| IBIS file stm32u073_083_ufqfpn48.ibs
[IBIS ver] 4.2
[File name] stm32u073_083_ufqfpn48.ibs
[File Rev] 0.3
[Date] 20-02-2024
[Source] Data Created at STMicroelectronics
[Notes]  File originated from ELDO simulations.
[Disclaimer]  This information is for modeling purpose only and is
   not guaranteed. The information is subject to change without
   notice.
[Copyright] Copyright 2024 STMicroelectronics Inc.
|   Component stm32u073_083_ufqfpn48
[Component] stm32u073_083_ufqfpn48
[Manufacturer] STMicroelectronics
[Package]
| variable   typ   min   max
R_pkg  0  NA  NA
L_pkg  0  NA  NA
C_pkg  0  NA  NA
[Pin]   signal_name   model_name
1  VBAT  power
2  PC13  io8_ft_v33
3  PC14-OSC32_IN  io8_ft_v33
4  PC15-OSC32_OUT  io8_ft
5  PF0-OSC_IN  io8_ft
6  PF1-OSC_OUT  io8_ft
7  PF2-NRST  ioreset_ft_v33
8  VSSA_VREFM  nc
9  VDDA_VREFP  nc
10  PA0  io8_ft_v33
11  PA1  io8_ft_v33
12  PA2  io8_ft_v33
13  PA3  io8_ft
14  PA4  io8_ft
15  PA5  io8_ft
16  PA6  io8_ft_i2c
17  PA7  io8_ft_i2c
18  PB0  io8_ft
19  PB1  io8_ft
20  PB2  io8_ft
21  PB10  io8_ft_i2c
22  PB11  io8_ft_i2c
23  VSS  gnd
24  VDD  power
25  PB12  io8_ft
26  PB13  io8_ft_i2c
27  PB14  io8_ft_i2c
28  PB15  io8_ft_v33
29  PA8  io8_ft
30  PA9  io8_ft_i2c
31  PA10  io8_ft_i2c
32  PA11  io8usb_ft_phy
33  PA12  io8usb_ft_phy
34  PA13  io8_ft
35  VSS  gnd
36  VDDUSB  power
37  PA14  io8_ft
38  PA15  io8_ft
39  PB3  io8_ft_i2c
40  PB4  io8_ft_i2c
41  PB5  io8_ft
42  PB6  io8_ft_i2c
43  PB7  io8_ft_i2c
44  PF3-BOOT0  io8_ft_v33
45  PB8  io8_ft_i2c
46  PB9  io8_ft_i2c
47  VSS  gnd
48  VDD  power
[Package Model]   489-qfpn-7x7-48-ldo-240125
[Pin Mapping]   pulldown_ref   pullup_ref   | Comment
1  nc  vsw
2  gndio  vddio  | Depending on IO usage
| 2  gndio  vsw  | Depending on IO usage
3  gndio  vddio  | Depending on IO usage
| 3  gndio  vsw  | Depending on IO usage
4  gndio  vddio  | Depending on IO usage
| 4  gndio  vsw  | Depending on IO usage
5  gndio  vddio
6  gndio  vddio
7  gndio  vddio
8  nc  nc
9  nc  nc
10  gndio  vddio
11  gndio  vddio
12  gndio  vddio
13  gndio  vddio
14  gndio  vddio
15  gndio  vddio
16  gndio  vddio
17  gndio  vddio
18  gndio  vddio
19  gndio  vddio
20  gndio  vddio
21  gndio  vddio
22  gndio  vddio
23  gndio  nc
24  nc  vddio
25  gndio  vddio
26  gndio  vddio
27  gndio  vddio
28  gndio  vddio
29  gndio  vddio
30  gndio  vddio
31  gndio  vddio
32  gndio  vddusb  | Depending on IO usage
| 32  gndio  vddio  | Depending on IO usage
33  gndio  vddusb  | Depending on IO usage
| 33  gndio  vddio  | Depending on IO usage
34  gndio  vddio
35  gndio  nc
36  nc  vddusb
37  gndio  vddio
38  gndio  vddio
39  gndio  vddio
40  gndio  vddio
41  gndio  vddio
42  gndio  vddio
43  gndio  vddio
44  gndio  vddio
45  gndio  vddio
46  gndio  vddio
47  gndio  nc
48  nc  vddio
|[Diff Pin]  inv_pin  vdiff  tdelay_typ  tdelay_min  tdelay_max
|33  32  NA  NA  NA  NA
[Model Selector] io8_ft
io8_ft_ls_1v2   "GPIO - 5V tolerant - 1.2V range - Low speed"
io8_ft_ms_1v2   "GPIO - 5V tolerant - 1.2V range - Med speed"
io8_ft_fs_1v2   "GPIO - 5V tolerant - 1.2V range - Fast speed"
io8_ft_hs_1v2   "GPIO - 5V tolerant - 1.2V range - High speed"
io8_ft_ls_1v8   "GPIO - 5V tolerant - 1.8V range - Low speed"
io8_ft_ms_1v8   "GPIO - 5V tolerant - 1.8V range - Med speed"
io8_ft_fs_1v8   "GPIO - 5V tolerant - 1.8V range - Fast speed"
io8_ft_hs_1v8   "GPIO - 5V tolerant - 1.8V range - High speed"
io8_ft_ls_3v3   "GPIO - 5V tolerant - 3.3V range - Low speed"
io8_ft_ms_3v3   "GPIO - 5V tolerant - 3.3V range - Med speed"
io8_ft_fs_3v3   "GPIO - 5V tolerant - 3.3V range - Fast speed"
io8_ft_hs_3v3   "GPIO - 5V tolerant - 3.3V range - High speed"
[Model Selector] io8_ft_i2c
io8_ft_ls_1v2   "GPIO - 5V tolerant - 1.2V range - Low speed"
io8_ft_ms_1v2   "GPIO - 5V tolerant - 1.2V range - Med speed"
io8_ft_fs_1v2   "GPIO - 5V tolerant - 1.2V range - Fast speed"
io8_ft_hs_1v2   "GPIO - 5V tolerant - 1.2V range - High speed"
io8_ft_ls_1v8   "GPIO - 5V tolerant - 1.8V range - Low speed"
io8_ft_ms_1v8   "GPIO - 5V tolerant - 1.8V range - Med speed"
io8_ft_fs_1v8   "GPIO - 5V tolerant - 1.8V range - Fast speed"
io8_ft_hs_1v8   "GPIO - 5V tolerant - 1.8V range - High speed"
io8_ft_ls_3v3   "GPIO - 5V tolerant - 3.3V range - Low speed"
io8_ft_ms_3v3   "GPIO - 5V tolerant - 3.3V range - Med speed"
io8_ft_fs_3v3   "GPIO - 5V tolerant - 3.3V range - Fast speed"
io8_ft_hs_3v3   "GPIO - 5V tolerant - 3.3V range - High speed"
io8_ft_i2c_ls_1v2   "GPIO I2C open-drain - 5V tolerant - 1.2V range - Low speed"
io8_ft_i2c_ms_1v2   "GPIO I2C open-drain - 5V tolerant - 1.2V range - Med speed"
io8_ft_i2c_fs_1v2   "GPIO I2C open-drain - 5V tolerant - 1.2V range - Fast speed"
io8_ft_i2c_hs_1v2   "GPIO I2C open-drain - 5V tolerant - 1.2V range - High speed"
io8_ft_i2c_ls_1v8   "GPIO I2C open-drain - 5V tolerant - 1.8V range - Low speed"
io8_ft_i2c_ms_1v8   "GPIO I2C open-drain - 5V tolerant - 1.8V range - Med speed"
io8_ft_i2c_fs_1v8   "GPIO I2C open-drain - 5V tolerant - 1.8V range - Fast speed"
io8_ft_i2c_hs_1v8   "GPIO I2C open-drain - 5V tolerant - 1.8V range - High speed"
io8_ft_i2c_ls_3v3   "GPIO I2C open-drain - 5V tolerant - 3.3V range - Low speed"
io8_ft_i2c_ms_3v3   "GPIO I2C open-drain - 5V tolerant - 3.3V range - Med speed"
io8_ft_i2c_fs_3v3   "GPIO I2C open-drain - 5V tolerant - 3.3V range - Fast speed"
io8_ft_i2c_hs_3v3   "GPIO I2C open-drain - 5V tolerant - 3.3V range - High speed"
io8_ft_i2c_fmp_3v3   "GPIO I2C open-drain fm+ - 5V tolerant - 3.3V range"
[Model Selector] io8_ft_v33
io8_ft_v33_ls_1v2   "GPIO_V33 - 5V tolerant - 1.2V range - Low speed"
io8_ft_v33_ms_1v2   "GPIO_V33 - 5V tolerant - 1.2V range - Med speed"
io8_ft_v33_fs_1v2   "GPIO_V33 - 5V tolerant - 1.2V range - Fast speed"
io8_ft_v33_hs_1v2   "GPIO_V33 - 5V tolerant - 1.2V range - High speed"
io8_ft_v33_ls_1v8   "GPIO_V33 - 5V tolerant - 1.8V range - Low speed"
io8_ft_v33_ms_1v8   "GPIO_V33 - 5V tolerant - 1.8V range - Med speed"
io8_ft_v33_fs_1v8   "GPIO_V33 - 5V tolerant - 1.8V range - Fast speed"
io8_ft_v33_hs_1v8   "GPIO_V33 - 5V tolerant - 1.8V range - High speed"
io8_ft_v33_ls_3v3   "GPIO_V33 - 5V tolerant - 3.3V range - Low speed"
io8_ft_v33_ms_3v3   "GPIO_V33 - 5V tolerant - 3.3V range - Med speed"
io8_ft_v33_fs_3v3   "GPIO_V33 - 5V tolerant - 3.3V range - Fast speed"
io8_ft_v33_hs_3v3   "GPIO_V33 - 5V tolerant - 3.3V range - High speed"
[Model Selector] io8usb_ft_phy
io8_ft_ls_1v2   "GPIO - 5V tolerant - 1.2V range - Low speed"
io8_ft_ms_1v2   "GPIO - 5V tolerant - 1.2V range - Med speed"
io8_ft_fs_1v2   "GPIO - 5V tolerant - 1.2V range - Fast speed"
io8_ft_hs_1v2   "GPIO - 5V tolerant - 1.2V range - High speed"
io8_ft_ls_1v8   "GPIO - 5V tolerant - 1.8V range - Low speed"
io8_ft_ms_1v8   "GPIO - 5V tolerant - 1.8V range - Med speed"
io8_ft_fs_1v8   "GPIO - 5V tolerant - 1.8V range - Fast speed"
io8_ft_hs_1v8   "GPIO - 5V tolerant - 1.8V range - High speed"
io8_ft_ls_3v3   "GPIO - 5V tolerant - 3.3V range - Low speed"
io8_ft_ms_3v3   "GPIO - 5V tolerant - 3.3V range - Med speed"
io8_ft_fs_3v3   "GPIO - 5V tolerant - 3.3V range - Fast speed"
io8_ft_hs_3v3   "GPIO - 5V tolerant - 3.3V range - High speed"
io8usb_ft_phy_hs_3v3   "USB full speed"
io8usb_ft_phy_ls_3v3   "USB low speed"
[Model Selector] ioreset_ft_v33
ioreset_ft_v33_1v2   "Reset PAD. 5V tolerant. 1.2V range"
ioreset_ft_v33_1v8   "Reset PAD. 5V tolerant. 1.8V range"
ioreset_ft_v33_3v3   "Reset PAD. 5V tolerant. 3.3V range"
[Define Package Model]  489-qfpn-7x7-48-ldo-240125
[Manufacturer]  Unknown
[OEM]  Unknown
[Description]  None
[Number Of Pins]  46
[Pin Numbers]
| Pin Num   Terminal Name
10 | PA0
11 | PA1
12 | PA2
13 | PA3
14 | PA4
15 | PA5
16 | PA6
17 | PA7
29 | PA8
30 | PA9
31 | PA10
32 | PA11
33 | PA12
34 | PA13
37 | PA14
38 | PA15
18 | PB0
19 | PB1
20 | PB2
39 | PB3
40 | PB4
41 | PB5
42 | PB6
43 | PB7
45 | PB8
46 | PB9
21 | PB10
22 | PB11
25 | PB12
26 | PB13
27 | PB14
28 | PB15
2 | PC13
3 | PC14-OSC32_IN
4 | PC15-OSC32_OUT
5 | PF0-OSC_IN
6 | PF1-OSC_OUT
7 | PF2-NRST
44 | PF3-BOOT0
1 | VBAT
48 | VDD
24 | VDD
9 | VDDA_VREFP
36 | VDDUSB
23 | VSS
8 | VSSA_VREFM
|[Merged Pins]  23
|35  |  VSS
|47  |  VSS
[Model Data]
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[End Model Data]
[End Package Model]
|End [Component]
| Models and submodels in the file (42): io8_ft_fs_1v2 (I/O), io8_ft_fs_1v8 (I/O), io8_ft_fs_3v3 (I/O), io8_ft_hs_1v2 (I/O), io8_ft_hs_1v8 (I/O), io8_ft_hs_3v3 (I/O), io8_ft_i2c_fmp_3v3 (I/O_open_drain), io8_ft_i2c_fs_1v2 (I/O_open_drain), io8_ft_i2c_fs_1v8 (I/O_open_drain), io8_ft_i2c_fs_3v3 (I/O_open_drain), io8_ft_i2c_hs_1v2 (I/O_open_drain), io8_ft_i2c_hs_1v8 (I/O_open_drain), io8_ft_i2c_hs_3v3 (I/O_open_drain), io8_ft_i2c_ls_1v2 (I/O_open_drain), io8_ft_i2c_ls_1v8 (I/O_open_drain), io8_ft_i2c_ls_3v3 (I/O_open_drain), io8_ft_i2c_ms_1v2 (I/O_open_drain), io8_ft_i2c_ms_1v8 (I/O_open_drain), io8_ft_i2c_ms_3v3 (I/O_open_drain), io8_ft_ls_1v2 (I/O), io8_ft_ls_1v8 (I/O), io8_ft_ls_3v3 (I/O), io8_ft_ms_1v2 (I/O), io8_ft_ms_1v8 (I/O), io8_ft_ms_3v3 (I/O), io8_ft_v33_fs_1v2 (I/O), io8_ft_v33_fs_1v8 (I/O), io8_ft_v33_fs_3v3 (I/O), io8_ft_v33_hs_1v2 (I/O), io8_ft_v33_hs_1v8 (I/O), io8_ft_v33_hs_3v3 (I/O), io8_ft_v33_ls_1v2 (I/O), io8_ft_v33_ls_1v8 (I/O), io8_ft_v33_ls_3v3 (I/O), io8_ft_v33_ms_1v2 (I/O), io8_ft_v33_ms_1v8 (I/O), io8_ft_v33_ms_3v3 (I/O), io8usb_ft_phy_hs_3v3 (I/O), io8usb_ft_phy_ls_3v3 (I/O), ioreset_ft_v33_1v2 (I/O_open_drain), ioreset_ft_v33_1v8 (I/O_open_drain), ioreset_ft_v33_3v3 (I/O_open_drain)
